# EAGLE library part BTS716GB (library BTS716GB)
BTS716GB Smart High-Side Power Switch, Four Channels: 4x140mOhm, Status Feedback, VBB 43V SOIC127P1030X265-20N-1
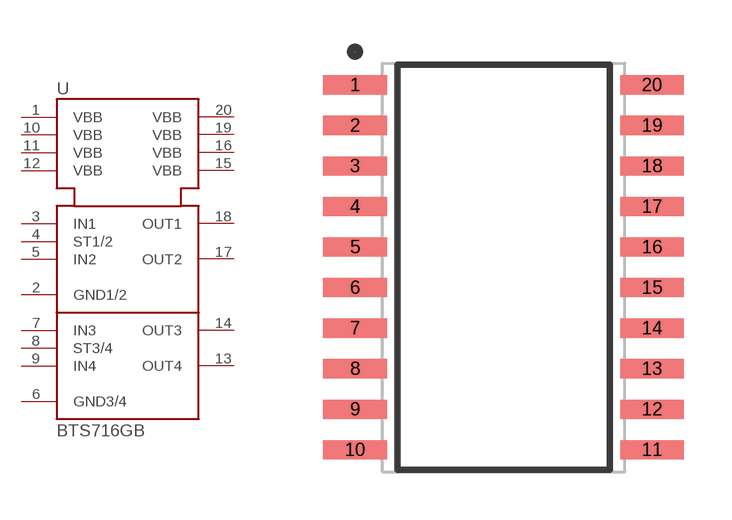
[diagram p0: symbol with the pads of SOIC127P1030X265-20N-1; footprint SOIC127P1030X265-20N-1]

Designator prefix U

## BTS716GB  [SOIC127P1030X265-20N-1]
1  VBB  pwr
2  GND1/2  pwr
3  IN1  in
4  ST1/2  oc
5  IN2  in
6  GND3/4  pwr
7  IN3  in
8  ST3/4  oc
9  IN4  in
10  VBB  pwr
11  VBB  pwr
12  VBB  pwr
13  OUT4  out
14  OUT3  out
15  VBB  pwr
16  VBB  pwr
17  OUT2  out
18  OUT1  out
19  VBB  pwr
20  VBB  pwr

## Footprint SOIC127P1030X265-20N-1 (pad centres in mm)
Original name SOIC127P1030X265-20N-1 Max Component Height - 2.65mm
smd 2 x 0.6: 1 -4.65,5.715; 2 -4.65,4.445; 3 -4.65,3.175; 4 -4.65,1.905; 5 -4.65,0.635; 6 -4.65,-0.635; 7 -4.65,-1.905; 8 -4.65,-3.175; 9 -4.65,-4.445; 10 -4.65,-5.715; 11 4.65,-5.715; 12 4.65,-4.445; 13 4.65,-3.175; 14 4.65,-1.905; 15 4.65,-0.635; 16 4.65,0.635; 17 4.65,1.905; 18 4.65,3.175; 19 4.65,4.445; 20 4.65,5.715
